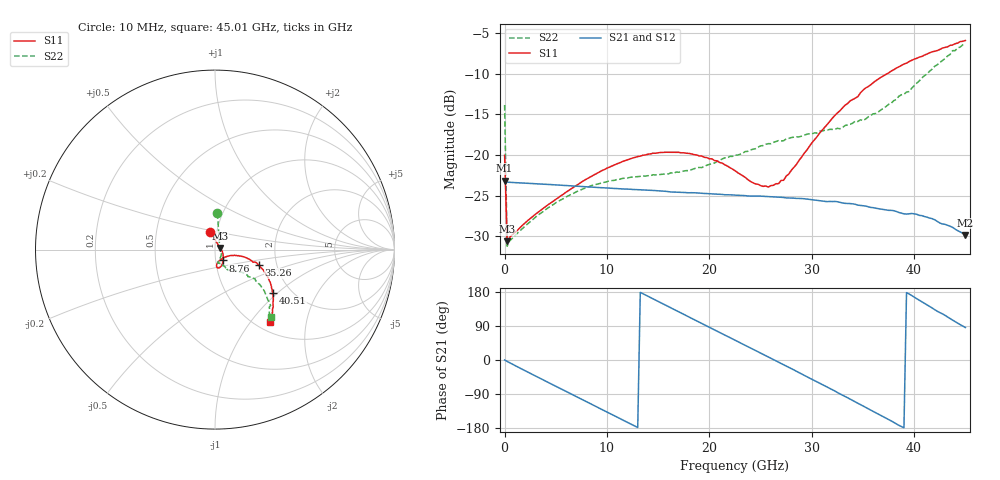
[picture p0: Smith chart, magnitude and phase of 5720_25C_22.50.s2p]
! Device:  ADRF5720
! Description: 0.5dB LSB GaAs MMIC 6-bit Digital Attenuator
! Frequency:  0.000009 -  40 GHz
! Ports:
!	RF1	= Port 1
!	RF2	= Port 2
! Vdd:  3.3 Volt
! Vss:  -3.3 Volt
! Control:  0/3.3 Volt
! State:  22.50 dB attenuation
! Data:  The device was measured using G-S-G Probes on a matrix board.
!  Data was collected using an calibrated 4 port network analyzer.
!  The reference plane for this measurement is at the launchers.
! Note:  Analog Devices supplies this data as a sample of measured data
!  for this product.  Your particular data for this product may vary.
!  Data was taken at 25 degrees C.
!  Analog Devices reserves the right to change this data at anytime.
# GHZ S DB R 45.0
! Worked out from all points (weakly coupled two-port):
!   181 points, 10 MHz to 45.01 GHz, reference 45 ohm
!   highest |S21| = -23.13 dB at 10 MHz (marker M1); lowest = -29.8 dB at 45.01 GHz (marker M2)
!   lowest |S11| = -30.6 dB at 260 MHz (marker M3), VSWR 1.06, Z = 47.6 + j0.862 ohm
!   |S11| at or under -10 dB: start of sweep to 37.35 GHz
!   |S22| runs from -31.2 to -6.2 dB; largest |S21 - S12| = 0.00017
!   S11 on the Smith chart (normalised r, x): 10 MHz: 0.93, +0.18; 8.76 GHz: 1.09, -0.13; 35.26 GHz: 1.61, -0.30; 40.51 GHz: 1.62, -0.92; 45.01 GHz: 1.15, -1.25
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0.01  -20.03 104.9  -23.13 0.1  -23.13 0.1  -13.83 86.2
0.26  -30.61 17.9  -23.33 -3.8  -23.33 -3.8  -31.21 17.0
0.51  -30.12 9.5  -23.35 -7.4  -23.35 -7.4  -30.54 6.9
3.26  -27.05 -18.9  -23.54 -45.5  -23.54 -45.4  -27.40 -34.0
7.76  -23.13 -48.1  -23.88 -106.7  -23.88 -106.7  -24.11 -67.0
8.760001  -22.43 -52.9  -23.96 -120.3  -23.95 -120.3  -23.67 -70.6
12.01  -20.57 -65.9  -24.19 -164.5  -24.19 -164.4  -22.82 -77.6
15.26  -19.67 -76.0  -24.41 150.9  -24.41 150.9  -22.38 -76.9
19.26  -20.11 -84.1  -24.70 96.5  -24.70 96.5  -21.54 -68.7
22.76  -22.15 -81.4  -24.94 48.9  -24.94 48.9  -20.00 -61.9
25.26  -23.85 -60.5  -25.07 14.8  -25.07 14.8  -18.82 -59.9
26.76  -23.52 -41.5  -25.18 -5.6  -25.18 -5.6  -18.22 -58.2
27.76  -22.34 -29.5  -25.28 -19.3  -25.29 -19.3  -17.94 -58.0
30.26  -18.13 -15.2  -25.52 -54.2  -25.52 -54.1  -17.27 -56.2
32.26  -15.13 -14.4  -25.70 -81.8  -25.70 -81.7  -16.84 -52.8
35.26  -11.75 -19.4  -26.27 -124.9  -26.28 -124.9  -15.57 -45.5
37.76  -9.66 -27.4  -26.80 -160.7  -26.80 -160.6  -13.63 -39.0
39.51  -8.49 -33.3  -27.22 174.2  -27.23 174.3  -12.18 -38.3
40.51  -7.94 -36.6  -27.42 157.7  -27.42 157.7  -10.87 -37.5
42.26  -7.13 -42.8  -28.16 128.8  -28.15 128.8  -8.89 -40.0
43.76  -6.45 -48.0  -28.89 105.2  -28.91 105.3  -7.14 -45.2
45.01  -5.89 -53.0  -29.83 85.6  -29.83 85.6  -6.25 -50.5
